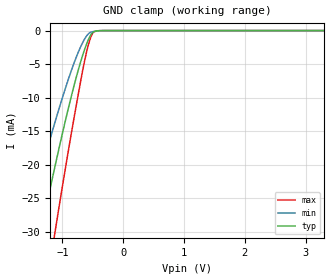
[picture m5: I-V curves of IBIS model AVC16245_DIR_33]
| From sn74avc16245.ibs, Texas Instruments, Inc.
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[Model]   AVC16245_DIR_33
Model_type  Input
Vinl = 0.8
Vinh = 2.0
| variable   typ   min   max
C_comp   2.03pF   1.47pF   2.38pF
[Temperature Range]   40   100   -40
| Ambient temperature   25   85   -40
[Voltage range]   3.3   3   3.6
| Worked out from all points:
|   GND clamp passes 1 mA (typ) near -0.56 V on its own axis
[GND Clamp]
| AVC16245_DIR_33
|   Voltage   I(typ)   I(min)   I(max)
-3.3V     -121mA     -90.61mA   -168.1mA
-1.61V    -41.38mA   -29.65mA   -59.22mA
-1.36V    -30.32mA   -21.25mA   -44.02mA
-1.32V    -28.59mA   -19.94mA   -41.64mA
-1.13V    -20.57mA   -13.9mA    -30.54mA
-1.095V   -19.14mA   -12.83mA   -28.54mA
-780mV    -7.233mA   -4.155mA   -11.56mA
-640mV    -2.948mA   -1.337mA   -4.735mA
-540mV    -738uA     -268.9uA   -1.157mA
-485mV    -176.3uA   -127.9uA   -215.4uA
-390mV    -15.74uA   -24.32uA   -8.777uA
3.3V      718.9pA    11.01nA    43.35pA
